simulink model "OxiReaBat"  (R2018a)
settings: Solver=VariableStepAuto  StartTime=0.0  StopTime=40  RelTol=1e-3
undefined symbols (not defined in the file): b3b57b55, b791, b944, cc0f, cf89edc882ae, d2f43f2bfe82, f9231dcf, OxiReaBat, sdiscope

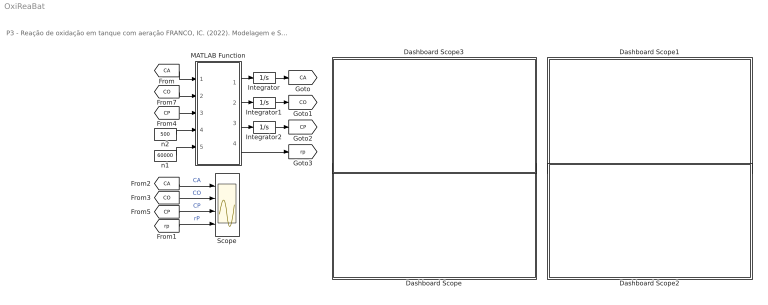
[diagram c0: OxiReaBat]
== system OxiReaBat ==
  note: P3 - Reação de oxidação em tanque com aeração FRANCO, IC. (2022). Modelagem e Simulação: Problemas Típicos da Engenharia Química para Simulação e Análise. NOTAS DE AULA INOVADORAS. The Journal of Engineering and Exact Sciences. Material Complementar.
  Dashboard Scope : Subsystem  DialogController=hmiCreateDDGDialog  IsWebBlock=on  mask(MWDashboardBlock){webBlockId=b3b57b55-9e5e-4329-8623-03168fabf3fe, webBlockType=sdiscope, ShowInitialText=on, HMISrcModelName=OxiReaBat}
      mask prompts: webBlockId "WebBlock Id"; webBlockType "WebBlock Type"; HMISrcModelName "Source Model"
      mask help: SimulinkHMI:dialogs:HMIScopeDialogDesc
  Dashboard Scope1 : Subsystem  DialogController=hmiCreateDDGDialog  IsWebBlock=on  mask(MWDashboardBlock){webBlockId=5c396c49-cc0f-4e77-8df0-cf89edc882ae, webBlockType=sdiscope, ShowInitialText=on, HMISrcModelName=OxiReaBat}
      mask prompts: webBlockId "WebBlock Id"; webBlockType "WebBlock Type"; HMISrcModelName "Source Model"
      mask help: SimulinkHMI:dialogs:HMIScopeDialogDesc
  Dashboard Scope2 : Subsystem  DialogController=hmiCreateDDGDialog  IsWebBlock=on  mask(MWDashboardBlock){webBlockId=f9231dcf-b944-4a72-b791-d2f43f2bfe82, webBlockType=sdiscope, ShowInitialText=on, HMISrcModelName=OxiReaBat}
      mask prompts: webBlockId "WebBlock Id"; webBlockType "WebBlock Type"; HMISrcModelName "Source Model"
      mask help: SimulinkHMI:dialogs:HMIScopeDialogDesc
  Dashboard Scope3 : Subsystem  DialogController=hmiCreateDDGDialog  IsWebBlock=on  mask(MWDashboardBlock){webBlockId=6421d89d-679e-4743-90bf-8c2659ef7523, webBlockType=sdiscope, ShowInitialText=on, HMISrcModelName=OxiReaBat}
      mask prompts: webBlockId "WebBlock Id"; webBlockType "WebBlock Type"; HMISrcModelName "Source Model"
      mask help: SimulinkHMI:dialogs:HMIScopeDialogDesc
  Integrator : Integrator  InitialCondition=0.2  LowerSaturationLimit=0
  Integrator1 : Integrator  LowerSaturationLimit=0
  Integrator2 : Integrator
  MATLAB Function : MATLAB Function  TreatAsAtomicUnit=on
  Scope : Scope  NumInputPorts=4
  n1 : Constant  Value=60000
  n2 : Constant  Value=500
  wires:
  MATLAB Function/1(dCA) -> Integrator/1
  Integrator/1 -> [CA]
  [CA] -> MATLAB Function/1(CA)
  [CA] -> Scope/1  "CA"
  [CO] -> Scope/2  "CO"
  Integrator1/1 -> [CO]
  MATLAB Function/2(dCO) -> Integrator1/1
  [CO] -> MATLAB Function/2(CO)
  MATLAB Function/4(rp) -> [rp]
  Integrator2/1 -> [CP]
  MATLAB Function/3(dCP) -> Integrator2/1
  [CP] -> MATLAB Function/3(CP)
  n2/1 -> MATLAB Function/4(N)
  [CP] -> Scope/3  "CP"
  [rp] -> Scope/4  "rP"
  n1/1 -> MATLAB Function/5(G)

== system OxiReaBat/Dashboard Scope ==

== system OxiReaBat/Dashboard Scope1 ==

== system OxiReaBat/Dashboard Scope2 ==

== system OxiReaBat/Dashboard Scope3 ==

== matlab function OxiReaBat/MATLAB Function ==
function [dCA,dCO,dCP,rp] = fcn(CA,CO,CP,N,G)
%% dados do processo
COs = 0.250e-3;
k   = 2.000e+3;
kt  = 0.900e-9;
%% equações auxiliares
rA = -k*CA*CO;
rO =  (1/2)*rA;
rp = -(1/2)*rA;
KLa= kt*N^3*G^0.5;

%% modelos matemáticos
dCA = rA;
dCO = KLa*(COs-CO)+rO;
dCP = rp;
end
